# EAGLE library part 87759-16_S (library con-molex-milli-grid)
HEADER
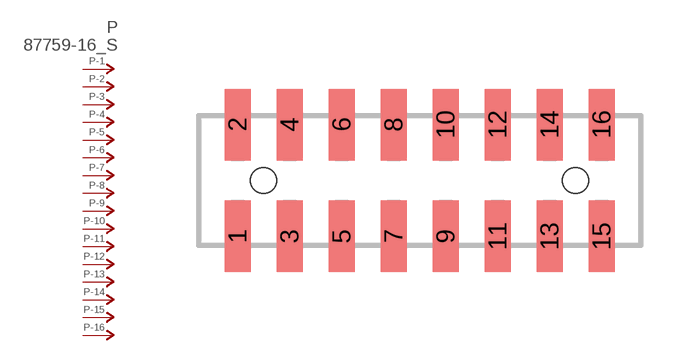
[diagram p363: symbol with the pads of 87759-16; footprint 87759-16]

Designator prefix P; gates -1=P-NV -2=P-N -3=P-N -4=P-N -5=P-N -6=P-N -7=P-N -8=P-N -9=P-N -10=P-N -11=P-N -12=P-N -13=P-N -14=P-N -15=P-N -16=P-N

## 87759-16_S  [87759-16]
1  -1:P  pas
2  -2:P  pas
3  -3:P  pas
4  -4:P  pas
5  -5:P  pas
6  -6:P  pas
7  -7:P  pas
8  -8:P  pas
9  -9:P  pas
10  -10:P  pas
11  -11:P  pas
12  -12:P  pas
13  -13:P  pas
14  -14:P  pas
15  -15:P  pas
16  -16:P  pas

## Footprint 87759-16 (pad centres in mm)
HEADER SMD Dual Row, Vertical
smd 1 x 2.75: 1 -7,-2.15; 2 -7,2.15; 3 -5,-2.15; 4 -5,2.15; 5 -3,-2.15; 6 -3,2.15; 7 -1,-2.15; 8 -1,2.15; 9 1,-2.15; 10 1,2.15; 11 3,-2.15; 12 3,2.15; 13 5,-2.15; 14 5,2.15; 15 7,-2.15; 16 7,2.15
hole 1 at -6,0
hole 1 at 6,0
